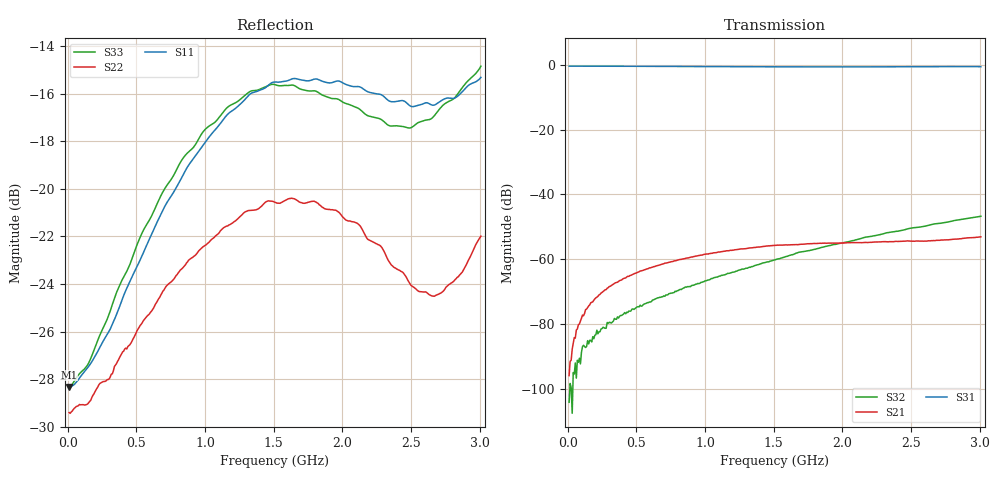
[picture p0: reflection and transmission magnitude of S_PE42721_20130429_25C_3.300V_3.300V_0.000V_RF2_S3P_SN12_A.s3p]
! Device ID: PE42721_20130429
! Serial: 12
! Insertion: A
! Temp: 25C
! VDD: 3.300
! Control_Hi: 3.300
! Control_Lo: 0.000
! Logic State: RF2
! ThroughPath: 3-1
! Port 1: RFC
! Port 2: RF1
! Port 3: RF2
! V1 = 3.30
! V2 = 0.00
! V3 = 0.00
! IDD: 1.093839e-04
! FILE NAME
! DATE 04-30-2013 12:04:22
! CORRECTED  DATA
#  Hz  S  RI  R  75
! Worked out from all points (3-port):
!   401 points, 10 MHz to 3.01 GHz, reference 75 ohm
!   strongest paths, dB at 10 MHz, 760 MHz, 1.51 GHz, 2.26 GHz, 3.01 GHz:
!     S31: -0.4, -0.5, -0.6, -0.6, -0.5
!     S21: -96.0, -60.8, -55.7, -54.7, -53.1
!     S32: -104.2, -70.5, -60.2, -52.6, -46.8
!   lowest |S11| = -28.3 dB at 10 MHz (marker M1), VSWR 1.08, Z = 81 - j0.196 ohm
!   |S11| at or under -10 dB: start of sweep to end of sweep
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1e7  0.0383 -0.00121  1.69e-06 5.63e-06  0.9555 -0.00217
     -8.23e-06 1.36e-05  0.0338 -0.00061  -1.66e-07 -1.37e-05
     0.9561 -0.00197  -3.55e-06 -5.01e-06  0.0381 -0.00145
7.75e7  0.0387 -0.00897  2.78e-06 9.8e-05  0.9551 -0.0161
        -3.13e-06 9.67e-05  0.0347 -0.0046  5.61e-07 -3.38e-05
        0.9558 -0.0159  -4.08e-07 -2.54e-05  0.0396 -0.00901
1.6e8  0.0383 -0.0188  -2.36e-06 0.000189  0.9543 -0.033
       6.28e-06 0.000196  0.0343 -0.00987  -1.62e-05 -5.19e-05
       0.955 -0.0328  -2.37e-05 -5.05e-05  0.0391 -0.019
2.95e8  0.0352 -0.0353  -7.76e-06 0.000364  0.9518 -0.0603
        -1.32e-05 0.000362  0.0356 -0.0177  -4.46e-05 -9.16e-05
        0.9525 -0.0601  -4.13e-05 -9.33e-05  0.0404 -0.0357
5.125e8  0.0252 -0.0647  -2.7e-05 0.000628  0.9456 -0.1037
         -2.78e-05 0.000628  0.0393 -0.0321  -0.000109 -0.000146
         0.9461 -0.103  -0.000106 -0.000151  0.0401 -0.0661
9.925e8  -0.00494 -0.1241  -9.18e-05 0.00117  0.9227 -0.1922
         -9.2e-05 0.00118  0.0512 -0.0559  -0.000338 -0.000294
         0.9239 -0.1922  -0.000338 -0.000296  0.0286 -0.1294
1.51e9  -0.0164 -0.167  -0.000169 0.00162  0.8908 -0.2802
        -0.000178 0.00162  0.065 -0.0674  -0.000789 -0.00056
        0.8923 -0.2797  -0.000795 -0.000563  -0.00625 -0.1656
1.96e9  -0.000815 -0.1686  -0.000341 0.00173  0.8609 -0.3529
        -0.000335 0.00174  0.0641 -0.063  -0.00148 -0.000831
        0.862 -0.3512  -0.00148 -0.000849  -0.042 -0.1489
2.6575e9  -0.0103 -0.1497  -0.000998 0.00164  0.8084 -0.4747
          -0.00101 0.00164  0.0153 -0.0575  -0.00317 -0.00135
          0.8103 -0.4733  -0.00317 -0.00134  -0.0809 -0.1157
3.01e9  -0.0726 -0.1555  -0.00159 0.00154  0.764 -0.5463
        -0.0016 0.00152  -0.0241 -0.0758  -0.00431 -0.0015
        0.7661 -0.5437  -0.00433 -0.00151  -0.1055 -0.1473
